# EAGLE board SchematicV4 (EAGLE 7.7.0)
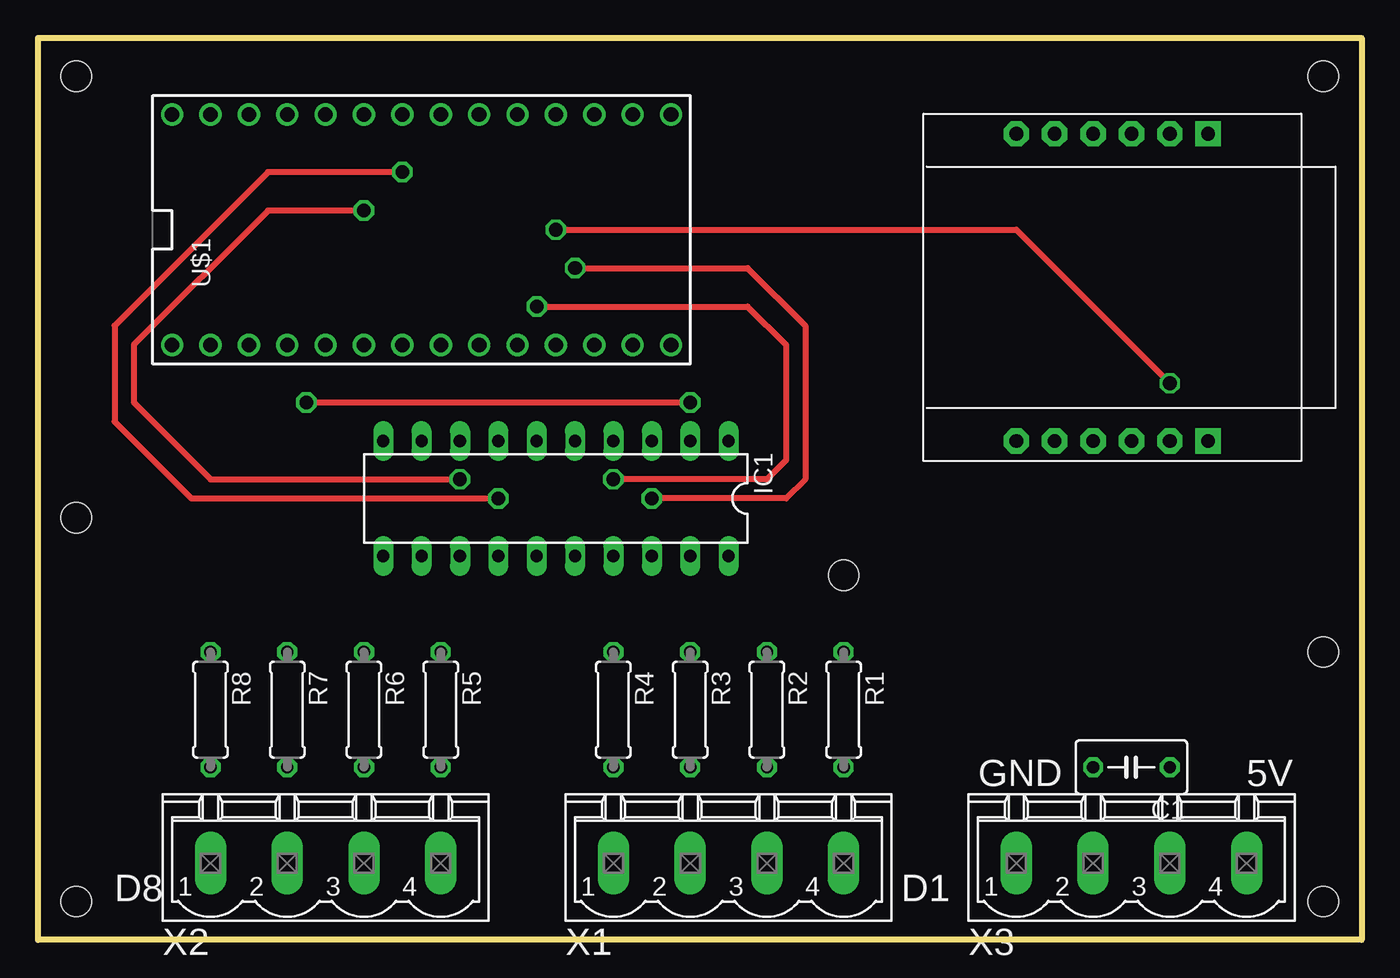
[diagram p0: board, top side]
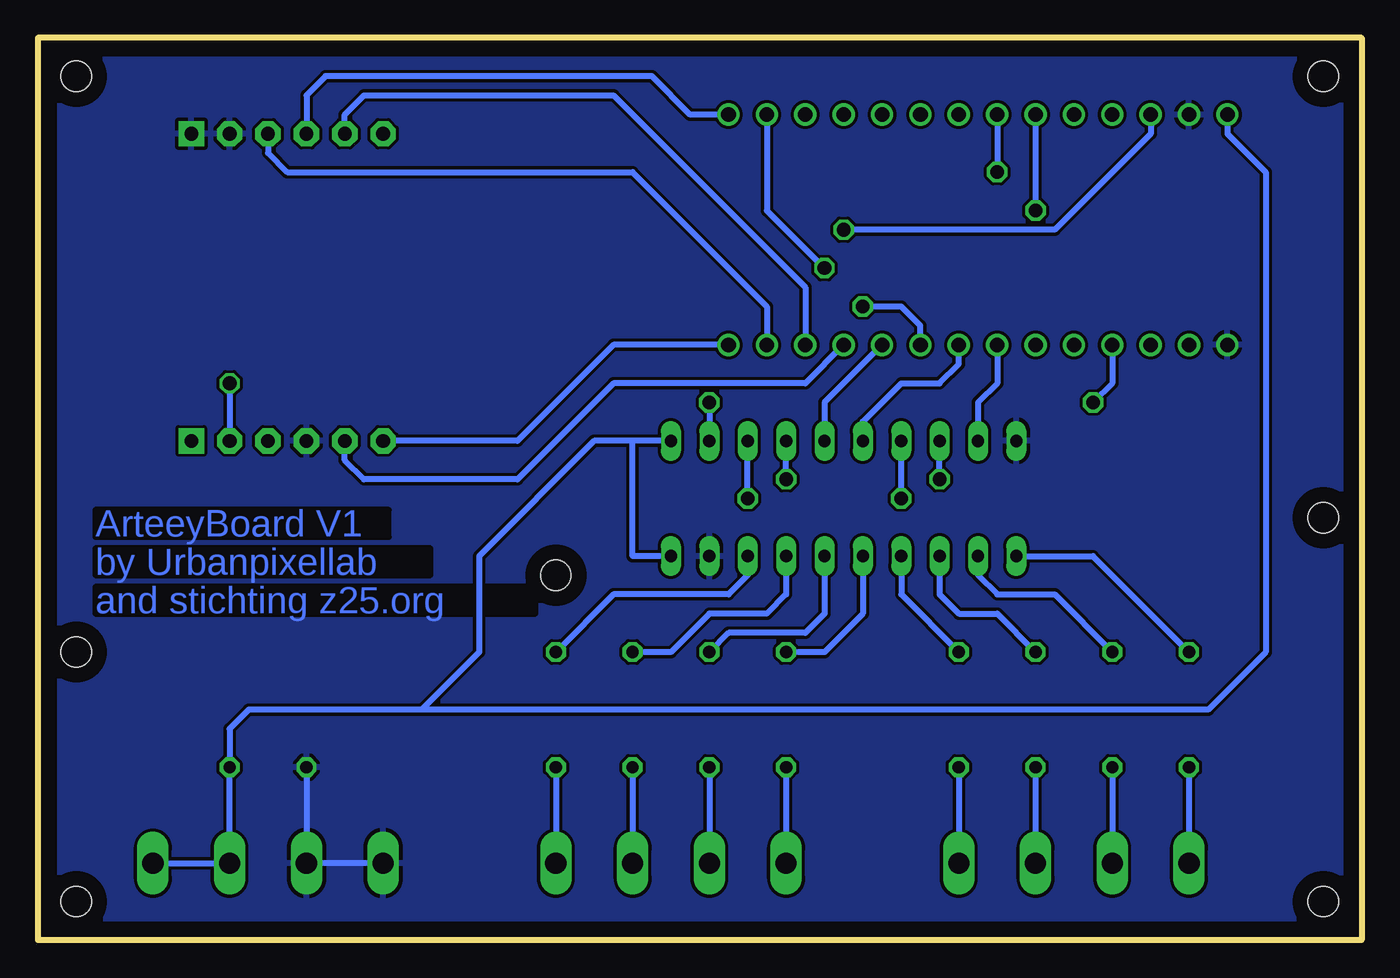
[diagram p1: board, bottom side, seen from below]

Size 87.63 x 59.69 mm. Coordinates in mm from the lower left corner, seen from the top.
Outline: 0,59.69 87.63,59.69 87.63,0 0,0 0,59.69
Copper layers (1*16): Top 0.035mm / dielectric 1.5mm / Bottom 0.035mm
Design rules "default": minimum track width 10mil, minimum drill 24mil, track to track 8mil, track to pad 8mil, pad to pad 8mil, via to via 8mil, smd to smd 8mil, copper to edge 40mil, drill to drill 8mil, minimum pad ring 10mil, minimum via ring 8mil, stop-mask expansion 4mil, vias tented up to drill 0mil, thermal gap 10mil
Holes 2 mm at 2.54,57.15 85.09,57.15 85.09,2.54 2.54,2.54 85.09,19.05 2.54,27.94 53.34,24.13

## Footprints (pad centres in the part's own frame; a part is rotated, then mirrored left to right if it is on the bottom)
C050-035X075 = drill 0.813 octagon: 1 -2.54,0; 2 2.54,0
DIL20 = drill 0.813 long: 1 -11.43,-3.81; 2 -8.89,-3.81; 3 -6.35,-3.81; 4 -3.81,-3.81; 5 -1.27,-3.81; 6 1.27,-3.81; 7 3.81,-3.81; 8 6.35,-3.81; 9 8.89,-3.81; 10 11.43,-3.81; 11 11.43,3.81; 12 8.89,3.81; 13 6.35,3.81; 14 3.81,3.81; 15 1.27,3.81; 16 -1.27,3.81; 17 -3.81,3.81; 18 -6.35,3.81; 19 -8.89,3.81; 20 -11.43,3.81
WIZ820IO = drill 0.9 pad 1.676 square: J1.1 -10.16,6.35; J2.1 10.16,6.35 | drill 0.9 pad 1.676 octagon: J1.2 -10.16,3.81; J1.3 -10.16,1.27; J1.4 -10.16,-1.27; J1.5 -10.16,-3.81; J1.6 -10.16,-6.35; J2.2 10.16,3.81; J2.3 10.16,1.27; J2.4 10.16,-1.27; J2.5 10.16,-3.81; J2.6 10.16,-6.35
0207/7 = drill 0.813 octagon: 1 -3.81,0; 2 3.81,0
TEENSY_3.0-3.2&LC_DIL = drill 0.965: 0 -7.62,13.97; 1 -7.62,11.43; 2 -7.62,8.89; 3 -7.62,6.35; 3.3V 7.62,11.43; 4 -7.62,3.81; 5 -7.62,1.27; 6 -7.62,-1.27; 7 -7.62,-3.81; 8 -7.62,-6.35; 9 -7.62,-8.89; 10 -7.62,-11.43; 11 -7.62,-13.97; 12 -7.62,-16.51; 13 7.62,-16.51; 14/A0 7.62,-13.97; 15/A1 7.62,-11.43; 16/A2 7.62,-8.89; 17/A3 7.62,-6.35; 18/A4 7.62,-3.81; 19/A5 7.62,-1.27; 20/A6 7.62,1.27; 21/A7 7.62,3.81; 22/A8 7.62,6.35; 23/A9 7.62,8.89; AGND 7.62,13.97; GND -7.62,16.51; VIN 7.62,16.51
MSTBV4 = drill 1.397 long: 1 -7.62,0; 2 -2.54,0; 3 2.54,0; 4 7.62,0

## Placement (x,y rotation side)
C1  1uF  [C050-035X075]  72.39,11.43 180 top
IC1  74LS245N  [DIL20]  34.29,29.21 180 top
IC2  WIZ820io  [WIZ820IO]  71.12,43.18 270 top
R1  100  [0207/7]  53.34,15.24 270 top
R2  100  [0207/7]  48.26,15.24 270 top
R3  100  [0207/7]  43.18,15.24 270 top
R4  100  [0207/7]  38.1,15.24 270 top
R5  100  [0207/7]  26.67,15.24 270 top
R6  100  [0207/7]  21.59,15.24 270 top
R7  100  [0207/7]  16.51,15.24 270 top
R8  100  [0207/7]  11.43,15.24 270 top
U$1  TEENSY_3.1-3.2_DIL  [TEENSY_3.0-3.2&LC_DIL]  25.4,46.99 90 top
X1  MSTBV4  [MSTBV4]  45.72,5.08 0 top
X2  MSTBV4  [MSTBV4]  19.05,5.08 0 top
X3  MSTBV4  [MSTBV4]  72.39,5.08 0 top

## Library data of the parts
C1 R1-R8 = resistor
IC1 = 74xx-us
IC2 = Wiz820io
U$1 = Teensy_3_and_LC_Series_Boards_v1.4
X1-X3 = con-phoenix-508; MPN: MSTBV 2,5/4-GF-5.08; OC_FARNELL: 1792794; OC_NEWARK: 69R9847

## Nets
+5V: C1.1 IC1.1 IC1.20 U$1.VIN X3.3 X3.4
GND: C1.2 IC1.10 IC1.19 IC2.J1.1 IC2.J1.2 IC2.J2.4 U$1.AGND U$1.GND X3.1 X3.2
GND3: IC2.J2.1
N$1: IC1.18 R1.1
N$2: IC1.17 R2.1
N$3: IC1.16 R3.1
N$4: IC1.15 R4.1
N$5: IC1.14 R5.1
N$6: IC1.13 R6.1
N$7: IC1.12 R7.1
N$8: IC1.11 R8.1
N$9: IC1.2 U$1.2
N$10: IC1.3 U$1.14/A0
N$11: IC1.4 U$1.7
N$12: IC1.5 U$1.8
N$13: IC1.6 U$1.6
N$14: IC1.7 U$1.20/A6
N$15: IC1.8 U$1.21/A7
N$16: IC1.9 U$1.5
N$18: IC2.J2.2 U$1.3.3V
N$19: IC2.J2.5 U$1.9
N$20: IC2.J2.6 U$1.12
N$21: IC2.J1.3 U$1.11
N$22: IC2.J1.4 U$1.13
N$23: IC2.J1.5 U$1.10
N$24: R1.2 X1.4
N$25: R2.2 X1.3
N$26: R3.2 X1.2
N$27: R4.2 X1.1
N$28: R5.2 X2.4
N$29: R6.2 X2.3
N$30: R7.2 X2.2
N$31: R8.2 X2.1
VIN2: IC2.J2.3

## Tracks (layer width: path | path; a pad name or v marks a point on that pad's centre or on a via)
+5V
  Bottom 0.406: X3.4 X3.3 C1.1 74.93,13.97 73.66,15.24 62.23,15.24 | U$1.VIN 8.89,53.34 6.35,50.8 6.35,19.05 10.16,15.24 62.23,15.24 | IC1.1 48.26,33.02 | 48.26,33.02 50.8,33.02 58.42,25.4 58.42,19.05 62.23,15.24 | IC1.20 48.26,25.4 48.26,33.02
GND
  Bottom 0.406: C1.2 X3.2 X3.1
  pour Bottom: 1.27,58.42 86.36,58.42 86.36,1.27 1.27,1.27
N$1
  Bottom 0.406: IC1.18 40.64,24.13 41.91,22.86 49.53,22.86 R1.1
N$2
  Bottom 0.406: IC1.17 38.1,22.86 39.37,21.59 43.18,21.59 45.72,19.05 R2.1
N$3
  Bottom 0.406: IC1.16 35.56,21.59 36.83,20.32 41.91,20.32 R3.1
N$4
  Bottom 0.406: IC1.15 33.02,21.59 35.56,19.05 R4.1
N$5
  Bottom 0.406: IC1.14 30.48,22.86 R5.1
N$6
  Bottom 0.406: IC1.13 27.94,22.86 26.67,21.59 24.13,21.59 R6.1
N$7
  Bottom 0.406: IC1.12 25.4,24.13 24.13,22.86 20.32,22.86 R7.1
N$8
  Bottom 0.406: IC1.11 17.78,25.4 R8.1
N$9  (via drill 0.9 pad 0.81)
  Top 0.406: v17.78,35.56 v43.18,35.56
  Bottom 0.406: U$1.2 16.51,36.83 v17.78,35.56 | v43.18,35.56 IC1.2
N$10  (via drill 0.9 pad 0.81)
  Top 0.406: v35.56,44.45 46.99,44.45 50.8,40.64 50.8,30.48 49.53,29.21 v40.64,29.21
  Bottom 0.406: U$1.14/A0 39.37,48.26 v35.56,44.45 | v40.64,29.21 IC1.3
N$11  (via drill 0.9 pad 0.81)
  Top 0.406: v33.02,41.91 46.99,41.91 49.53,39.37 49.53,31.75 48.26,30.48 v38.1,30.48
  Bottom 0.406: U$1.7 29.21,40.64 30.48,41.91 v33.02,41.91 | v38.1,30.48 IC1.4
N$12
  Bottom 0.406: U$1.8 35.56,35.56 IC1.5
N$13
  Bottom 0.406: IC1.6 33.02,34.29 30.48,36.83 27.94,36.83 26.67,38.1 U$1.6
N$14  (via drill 0.9 pad 0.81)
  Top 0.406: v24.13,50.8 15.24,50.8 5.08,40.64 5.08,34.29 10.16,29.21 v30.48,29.21
  Bottom 0.406: U$1.20/A6 v24.13,50.8 | v30.48,29.21 IC1.7
N$15  (via drill 0.9 pad 0.81)
  Top 0.406: v21.59,48.26 15.24,48.26 6.35,39.37 6.35,35.56 11.43,30.48 v27.94,30.48
  Bottom 0.406: U$1.21/A7 v21.59,48.26 | v27.94,30.48 IC1.8
N$16
  Bottom 0.406: U$1.5 24.13,36.83 25.4,35.56 IC1.9
N$18  (via drill 0.9 pad 0.81)
  Top 0.406: v34.29,46.99 64.77,46.99 v74.93,36.83
  Bottom 0.406: U$1.3.3V 13.97,53.34 20.32,46.99 v34.29,46.99 | v74.93,36.83 IC2.J2.2
N$19
  Bottom 0.406: U$1.9 36.83,36.83 49.53,36.83 55.88,30.48 66.04,30.48 67.31,31.75 IC2.J2.5
N$20
  Bottom 0.406: U$1.12 49.53,39.37 55.88,33.02 IC2.J2.6
N$21
  Bottom 0.406: IC2.J1.3 72.39,52.07 71.12,50.8 48.26,50.8 39.37,41.91 U$1.11
N$22
  Bottom 0.406: U$1.13 44.45,54.61 46.99,57.15 68.58,57.15 69.85,55.88 IC2.J1.4
N$23
  Bottom 0.406: IC2.J1.5 67.31,54.61 66.04,55.88 49.53,55.88 36.83,43.18 U$1.10
N$24
  Bottom 0.406: R1.2 X1.4
N$25
  Bottom 0.406: R2.2 X1.3
N$26
  Bottom 0.406: R3.2 X1.2
N$27
  Bottom 0.406: R4.2 X1.1
N$28
  Bottom 0.406: R5.2 X2.4
N$29
  Bottom 0.406: R6.2 X2.3
N$30
  Bottom 0.406: R7.2 X2.2
N$31
  Bottom 0.406: R8.2 X2.1

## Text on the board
Bottom: ArteeyBoard V1 | by Urbanpixellab | and stichting z25.org
tNames: GND | 5V | D8 | D1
